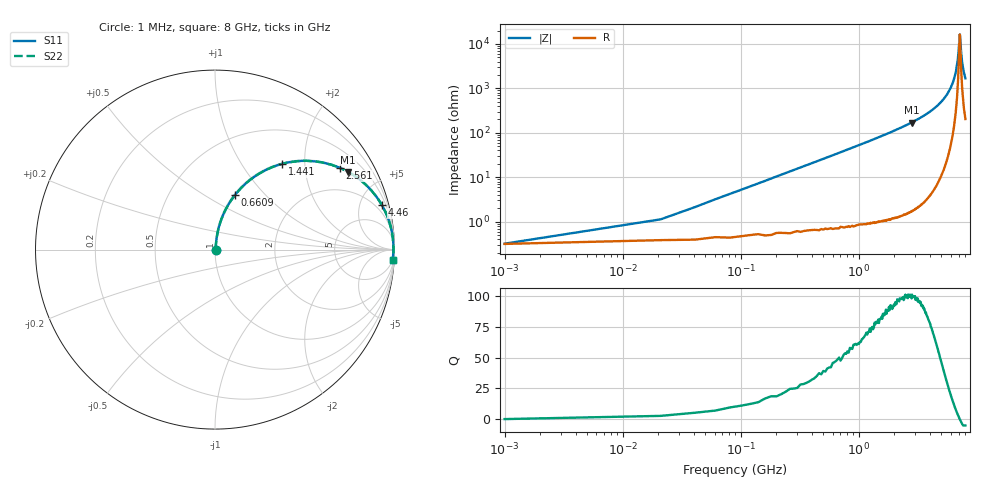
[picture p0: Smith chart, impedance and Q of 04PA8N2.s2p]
! Coilcraft 0402PA-8N2 Chip Inductor
! 11 March 2004
# MHZ S MA R 50
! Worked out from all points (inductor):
!   401 points, 1 MHz to 8 GHz, reference 50 ohm
!   read as one part in series: L = 8.22 nH near 40.99 MHz
!   highest Q = 99.9 at 2.801 GHz (marker M1), where L = 9.67 nH
!   self-resonance near 7.16 GHz
!   S11 on the Smith chart (normalised r, x): 1 MHz: 1.01, +0.00; 660.9 MHz: 1.01, +0.69; 1.441 GHz: 1.02, +1.55; 2.561 GHz: 1.03, +3.02; 4.46 GHz: 1.13, +7.49; 8 GHz: 5, -33
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1  0.003322 8.9  0.997 -0.0  0.997 -0.0  0.003322 8.9
60.992  0.032 80.3  0.995 -1.8  0.995 -1.8  0.032 80.3
80.99  0.042 81.4  0.995 -2.4  0.995 -2.4  0.042 81.4
160.98  0.082 81.7  0.992 -4.7  0.992 -4.7  0.082 81.7
360.955  0.182 77.6  0.977 -10.5  0.977 -10.5  0.182 77.6
660.917  0.323 70.0  0.94 -18.8  0.94 -18.8  0.323 70.0
1340.832  0.578 53.9  0.808 -35.3  0.808 -35.3  0.578 53.9
1440.82  0.608 51.8  0.786 -37.5  0.786 -37.5  0.608 51.8
2560.68  0.83 33.3  0.549 -56.1  0.549 -56.1  0.83 33.3
2680.665  0.845 31.8  0.526 -57.7  0.526 -57.7  0.845 31.8
2800.65  0.858 30.3  0.504 -59.1  0.504 -59.1  0.858 30.3
4000.5  0.945 18.4  0.316 -70.8  0.316 -70.8  0.945 18.4
4460.442  0.962 14.9  0.257 -74.2  0.257 -74.2  0.962 14.9
5340.333  0.983 9.2  0.159 -79.3  0.159 -79.3  0.983 9.2
6140.233  0.991 4.8  0.084 -81.8  0.084 -81.8  0.991 4.8
6680.165  0.994 2.2  0.039 -79.7  0.039 -79.7  0.994 2.2
6900.138  0.994 1.2  0.022 -73.6  0.022 -73.6  0.994 1.2
7140.108  0.994 0.2  0.006614 -24.2  0.006614 -24.2  0.994 0.2
7180.103  0.994 -0.0  0.006077 2.5  0.006077 2.5  0.994 -0.0
7380.078  0.994 -0.9  0.016 66.3  0.016 66.3  0.994 -0.9
7520.06  0.993 -1.4  0.026 74.1  0.026 74.1  0.993 -1.4
8000  0.991 -3.3  0.059 79.7  0.059 79.7  0.991 -3.3
